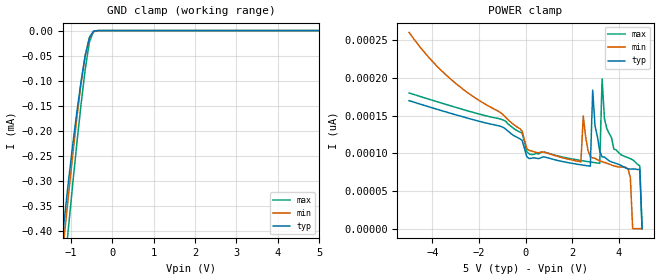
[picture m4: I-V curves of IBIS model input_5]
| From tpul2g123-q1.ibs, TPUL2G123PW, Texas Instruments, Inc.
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|   Model input_5
[Model] input_5
Model_type Input
Polarity   Non-Inverting
Enable   Active-High
Vinl =  0.0V
Vinh =  5.000V
C_comp   59.593fF   54.575fF   64.692fF
[Model Spec]
Vinh   5.000V   4.500V   5.500V
Vinl   0.0V   0.0V   0.0V
[Temperature Range]   27.000   0.125k   -40.000
[Voltage Range]   5.000V   4.500V   5.500V
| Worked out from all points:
|   GND clamp passes 1 mA (typ) near -1.86 V on its own axis
[GND_clamp]
|Voltage   I(typ)   I(min)   I(max)
-5V       -4.062mA   -3.727mA   -4.623mA
-1.263V   -457.4uA   -490.7uA   -567.3uA
-1.162V   -375.6uA   -408.1uA   -478.9uA
-1.061V   -299.3uA   -327.1uA   -391.5uA
-960mV    -227.8uA   -248.4uA   -306.4uA
-859mV    -161.8uA   -173.4uA   -224.4uA
-758mV    -101.4uA   -105.1uA   -147uA
-657mV    -49.68uA   -49.59uA   -77.18uA
-556mV    -13.85uA   -14.75uA   -22.67uA
-455mV    -1.126uA   -2.22uA    -1.283uA
-253mV    -759.1pA   -12.42nA   -5.639pA
5V        0A         0A         0A
[POWER_clamp]
|Voltage   I(typ)   I(min)   I(max)
-5V       169.9pA    260.6pA    180.1pA
152mV     93.06pA    103.8pA    99.2pA
2.374V    84.79pA    88.75pA    90.52pA
2.475V    84.31pA    149.6pA    90pA
2.778V    82.95pA    95.48pA    88.52pA
2.879V    184pA      94.04pA    88.05pA
3.182V    102.9pA    89.97pA    86.71pA
3.283V    95.29pA    88.88pA    198.8pA
3.788V    87.59pA    83.36pA    105.7pA
4.394V    79.41pA    79.14pA    94.27pA
4.899V    78.95pA    0A         83.43pA
5V        0A         0A         0A
